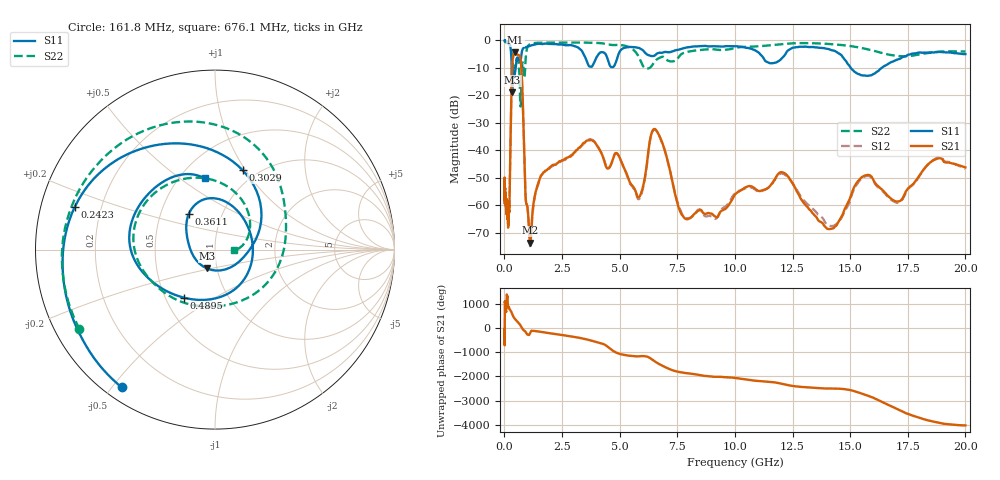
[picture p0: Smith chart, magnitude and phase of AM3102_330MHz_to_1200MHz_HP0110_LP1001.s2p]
! Date/Time: Tue, Sep 11, 2018 5:15 PM
! Network Analyzer: Agilent Technologies E8362B Rev: A.07.50.63
! Sweep from 0.010 to 20.000 GHz, 1601 Points, Sweep Type: LOG
! Power Supply: 4.949 V, 0.001 A
# Hz S DB R 50
!freq MagS11 AngS11 MagS21 AngS21 MagS12 AngS12 MagS22 AngS22
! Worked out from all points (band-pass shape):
!   1601 points, 10 MHz to 20 GHz, reference 50 ohm
!   highest |S21| = -4.28 dB at 469 MHz (marker M1); lowest = -73.6 dB at 1.119 GHz (marker M2)
!   |S21| within 3 dB of the highest: 355.9 MHz to 708.1 MHz (352.2 MHz wide, 66.2 % of centre)
!   lowest |S11| = -18.8 dB at 337.9 MHz (marker M3), VSWR 1.26, Z = 44.8 - j9.55 ohm
!   |S11| at or under -10 dB: 314.9 MHz to 488.6 MHz (173.7 MHz wide, 43.2 % of centre); 15.03 GHz to 16.37 GHz (1.346 GHz wide, 8.57 % of centre)
!   |S22| runs from -24.1 to -0.3 dB; largest |S21 - S12| = 0.011
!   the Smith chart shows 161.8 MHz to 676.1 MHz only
!   S11 on the Smith chart (normalised r, x): 161.8 MHz: 0.05, -0.53; 242.3 MHz: 0.10, +0.15; 302.9 MHz: 0.85, +0.97; 361.1 MHz: 0.69, +0.30; 489.5 MHz: 0.62, -0.37; 676.1 MHz: 0.66, +0.63
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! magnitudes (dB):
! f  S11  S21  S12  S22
! 10 MHz  0.0  -54.8  -51.5  -0.3
! 35.55 MHz  0.0  -57.6  -57.0  -0.5
! 126.4 MHz  -0.4  -64.9  -62.7  -1.0
! 161.8 MHz  -0.7  -68.1  -66.0  -1.2
! 242.3 MHz  -1.8  -48.9  -49.3  -1.8
! 302.9 MHz  -6.6  -20.0  -20.1  -3.4
! 337.9 MHz  -18.8  -9.5  -9.5  -6.5
! 361.1 MHz  -12.1  -6.9  -7.0  -8.2
! 447.2 MHz  -12.6  -4.3  -4.4  -9.4
! 469 MHz  -11.4  -4.3  -4.3  -8.7
! 489.5 MHz  -9.9  -4.3  -4.4  -8.0
! 676.1 MHz  -7.9  -5.9  -5.9  -19.3
! 1.119 GHz  -1.9  -73.6  -74.8  -1.3
! 1.59 GHz  -1.3  -49.2  -49.3  -0.8
! 3.739 GHz  -9.6  -36.3  -36.0  -0.8
! 5.652 GHz  -2.5  -54.1  -54.5  -3.9
! 6.549 GHz  -5.3  -32.4  -32.5  -7.4
! 7.92 GHz  -2.5  -65.1  -64.8  -4.2
! 12.03 GHz  -6.6  -48.0  -48.4  -1.4
! 14.14 GHz  -3.4  -68.6  -67.6  -1.3
! 15.55 GHz  -12.7  -49.6  -50.0  -2.8
! 20 GHz  -5.0  -46.2  -46.8  -4.1
